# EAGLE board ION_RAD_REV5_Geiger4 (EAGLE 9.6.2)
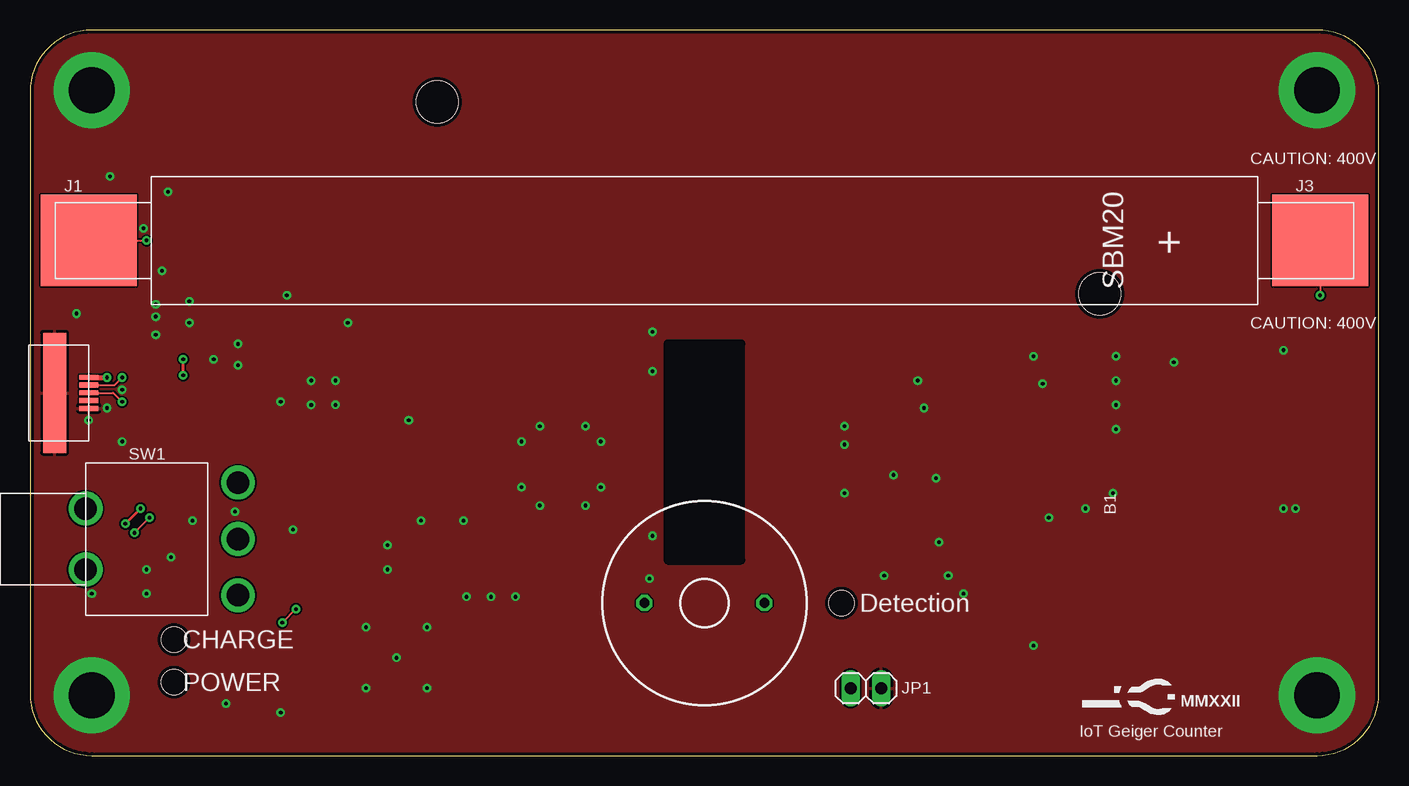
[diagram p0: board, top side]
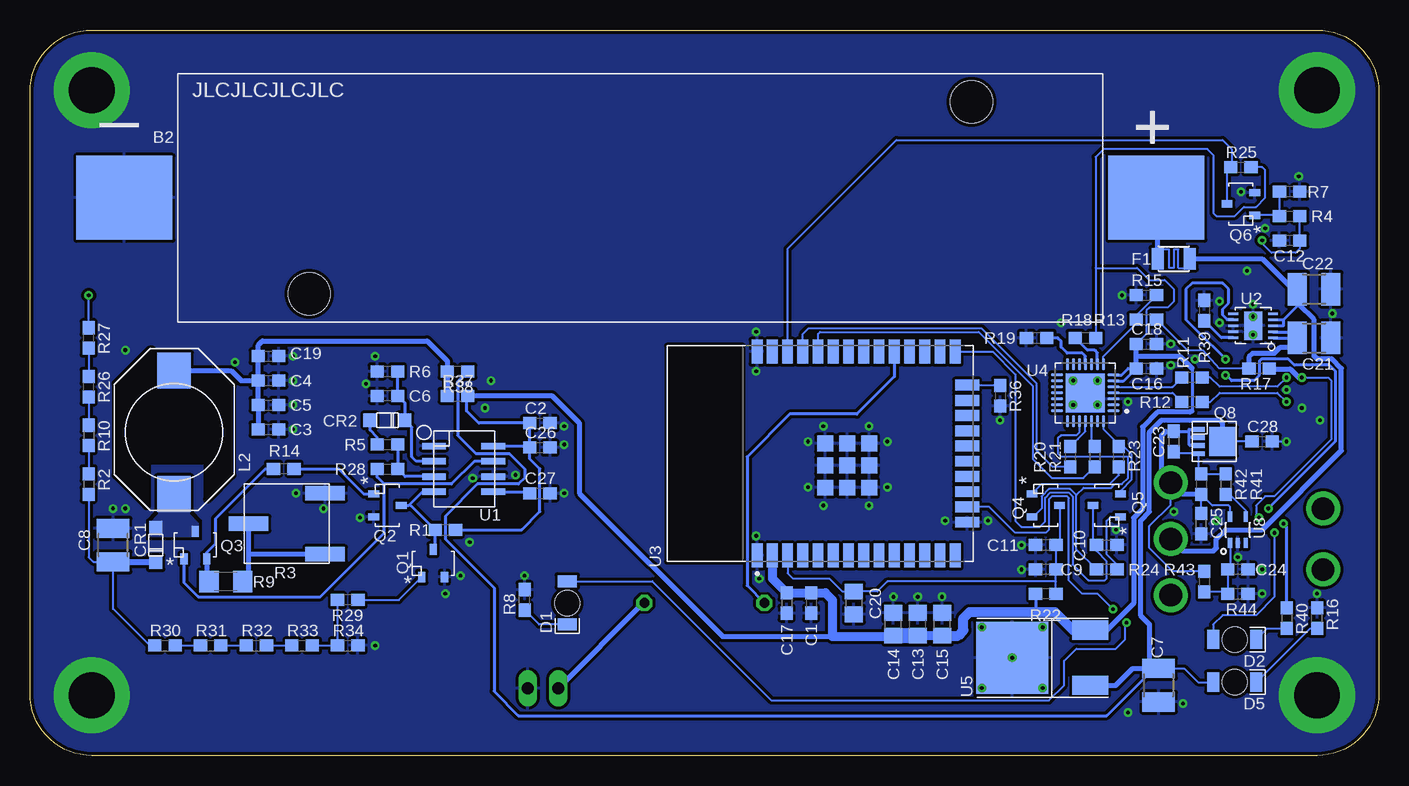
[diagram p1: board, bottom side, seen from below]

Size 112.4 x 60.5 mm. Coordinates in mm from the lower left corner, seen from the top.
Outline: 0,55.35 0,5.15 arc90 5.15,0 107.25,0 arc90 112.4,5.15 112.4,55.35 arc90 107.25,60.5 5.15,60.5 arc90 0,55.35
Copper layers (1*16): Top 0.035mm / dielectric 1.5mm / Bottom 0.035mm
Design rules "default *": minimum track width 6mil, minimum drill 12mil, track to track 6mil, track to pad 6mil, pad to pad 6mil, via to via 6mil, smd to smd 6mil, copper to edge 0.3mm, drill to drill 6mil, minimum pad ring 10mil, minimum via ring 8mil, stop-mask expansion 4mil, vias tented up to drill 12mil, thermal gap 10mil
Net classes: 1 HV: clearance 1.27 mm
tRestrict: area 53.2,16.3 to 59.2,34.3
bRestrict: area 95.6,20.9 to 105.2,33.8

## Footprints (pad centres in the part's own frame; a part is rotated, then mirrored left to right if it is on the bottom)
PS1740P02E = drill 0.813 octagon: 1 -5,0; 2 5,0
1042 = smd 8 x 7: + 43,0; - -43,0 | hole 3.5: -27.6,-8; 27.6,8
0603 = smd 1.1 x 1: 1 -0.85,0; 2 0.85,0
1210 = smd 1.6 x 2.7: 1 -1.4,0; 2 1.4,0
0805 = smd 1.3 x 1.5: 1 -0.95,0; 2 0.95,0
SOD123(AK) = smd 1.1 x 1.1: A 1.45,0; K -1.45,0
SOD123 = smd 1.1 x 1.1: 1 -1.45,0; 2 1.45,0
1206_REV = smd 1 x 1.6: A -1.8,0; K 1.8,0 | hole 2.1: 0,0
1206_FUSE_6M2_SS = smd 1.016 x 1.778: P$1 -1.333,0; P$2 1.333,0
01010002Z = smd 8.001 x 7.62: P$1 0,0
MICRO_USB = smd 0.4 x 1.6: 1 -1.3,0; 2 -0.65,0; 3 0,0; 4 0.65,0; 5 1.3,0 | smd 10 x 1.9: GND 0,-2.84
1X02 = drill 1.016 long: 1 -1.27,0; 2 1.27,0
SDR1005 = smd 3 x 2.8: P$1 -5.15,0; P$2 5.15,0
SOT23-3 = smd 0.6 x 0.9: 1 0.32,-1.15; 2 2.22,-1.15; 3 1.27,1.15
POWERPAK_1212-8 = smd 0.991 x 0.406: 1 -1.994,1.016; 2 -1.994,0.339; 3 -1.994,-0.339; 4 -1.994,-1.016 | smd 2.235 x 2.388: 15 0,0
3361P = smd 1.194 x 3.302: 1 -2.54,-3.188; 2 0,3.188; 3 2.54,-3.188
1206 = smd 1.6 x 1.8: 1 -1.4,0; 2 1.4,0
TOGGLE_RA = drill 1.88: 1 4.699,12.7; 2 0,12.7; 3 -4.699,12.7; P$4 -2.54,0; P$5 2.54,0
SOIC8 = smd 1.981 x 0.533: 1 -2.477,1.905; 2 -2.477,0.635; 3 -2.477,-0.635; 4 -2.477,-1.905; 5 2.477,-1.905; 6 2.477,-0.635; 7 2.477,0.635; 8 2.477,1.905
10DFN = smd 0.8 x 0.24: 1 -1.65,1; 2 -1.65,0.5; 3 -1.65,0; 4 -1.65,-0.5; 5 -1.65,-1; 6 1.65,-1; 7 1.65,-0.5; 8 1.65,0; 9 1.65,0.5; 10 1.65,1 | smd 1.5 x 2.4: GF 0,0
MODULE_ESP32-WROOM-32D = smd 2 x 0.9: 1 -8.5,5.26; 2 -8.5,3.99; 3 -8.5,2.72; 4 -8.5,1.45; 5 -8.5,0.18; 6 -8.5,-1.09; 7 -8.5,-2.36; 8 -8.5,-3.63; 9 -8.5,-4.9; 10 -8.5,-6.17; 11 -8.5,-7.44; 12 -8.5,-8.71; 13 -8.5,-9.98; 14 -8.5,-11.25; 25 8.5,-11.25; 26 8.5,-9.98; 27 8.5,-8.71; 28 8.5,-7.44; 29 8.5,-6.17; 30 8.5,-4.9; 31 8.5,-3.63; 32 8.5,-2.36; 33 8.5,-1.09; 34 8.5,0.18; 35 8.5,1.45; 36 8.5,2.72; 37 8.5,3.99; 38 8.5,5.26 | smd 0.9 x 2: 15 -5.715,-12.25; 16 -4.445,-12.25; 17 -3.175,-12.25; 18 -1.905,-12.25; 19 -0.635,-12.25; 20 0.635,-12.25; 21 1.905,-12.25; 22 3.175,-12.25; 23 4.445,-12.25; 24 5.715,-12.25 | smd 1.33 x 1.33: 39_1 -2.835,-0.405; 39_2 -1,-0.405; 39_3 0.835,-0.405; 39_4 -2.835,-2.24; 39_5 -1,-2.24; 39_6 0.835,-2.24; 39_7 -2.835,-4.075; 39_8 -1,-4.075; 39_9 0.835,-4.075
QFN50P500X500X80-29N = smd 1.01 x 0.27: 1 -2.36,1.5; 2 -2.36,1; 3 -2.36,0.5; 4 -2.36,0; 5 -2.36,-0.5; 6 -2.36,-1; 7 -2.36,-1.5; 15 2.36,-1.5; 16 2.36,-1; 17 2.36,-0.5; 18 2.36,0; 19 2.36,0.5; 20 2.36,1; 21 2.36,1.5 | smd 0.27 x 1.01: 8 -1.5,-2.36; 9 -1,-2.36; 10 -0.5,-2.36; 11 0,-2.36; 12 0.5,-2.36; 13 1,-2.36; 14 1.5,-2.36; 22 1.5,2.36; 23 1,2.36; 24 0.5,2.36; 25 0,2.36; 26 -0.5,2.36; 27 -1,2.36; 28 -1.5,2.36 | smd 3.25 x 3.25: 29 0,0
TO-252 = smd 1.6 x 3: 1 -2.3,-6.5; 3 2.3,-6.5 | smd 6 x 6: T 0,0
SC-70-5 = smd 0.85 x 0.35: 1 -1.1,0.65; 2 -1.1,0; 3 -1.1,-0.65; 4 1.1,-0.65; 5 1.1,0.65

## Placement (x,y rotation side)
B1  [PS1740P02E]  56.2,12.72 0 top
B2  1042  [1042]  61.53,46.51 0 bottom
C1  0.1uF  [0603]  47.31,12.72 270 bottom
C2  0.1uF  [0603]  69.92,27.71 0 bottom
C3  1uF  [0603]  92.52,27.2 0 bottom
C4  0.1uF  [0603]  92.52,31.27 0 bottom
C5  1uF  [0603]  92.52,29.23 0 bottom
C6  1nF  [0603]  82.62,30 180 bottom
C7  10uF  [1210]  18.35,5.87 270 bottom
C8  10nF 630V  [1210]  105.48,17.55 90 bottom
C9  0.1uF  [0603]  27.75,15.52 180 bottom
C10  0.1uF  [0603]  22.67,17.55 0 bottom
C11  0.1uF  [0603]  27.75,17.55 180 bottom
C12  100pF  [0603]  7.43,42.95 180 bottom
C13  10uF  [0805]  38.42,10.95 90 bottom
C14  1uF  [0805]  40.45,10.95 90 bottom
C15  1uF  [0805]  36.39,10.95 90 bottom
C16  0.1uF  [0603]  19.37,32.28 0 bottom
C17  0.1uF  [0603]  49.34,12.72 270 bottom
C18  0.1uF  [0603]  19.37,34.31 0 bottom
C19  1uF  [0603]  92.52,33.3 0 bottom
C20  10uF  [0805]  43.75,12.72 270 bottom
C21  4.7uF  [1210]  5.4,34.82 0 bottom
C22  4.7uF  [1210]  5.4,38.89 0 bottom
C23  0.1uF  [0603]  17.08,26.19 270 bottom
C24  0.1uF  [0603]  11.75,15.52 180 bottom
C25  0.1uF  [0603]  14.8,19.33 90 bottom
C26  0.1uF  [0603]  69.92,25.68 0 bottom
C27  0.1uF  [0603]  69.92,21.87 0 bottom
C28  0.1uF  [0603]  9.72,26.19 0 bottom
CR1  ES1JFL  [SOD123(AK)]  101.92,17.55 90 bottom
CR2  BAS21GWX  [SOD123]  82.62,27.96 180 bottom
D1  156120RS75300  [1206_REV]  67.63,12.72 270 bottom
D2  156120RS75300  [1206_REV]  12,9.68 0 bottom
D5  156120RS75300  [1206_REV]  12,6.12 0 bottom
F1  1206_FUSE6M2SS  [1206_FUSE_6M2_SS]  17.08,41.43 0 bottom
J1  01010002Z  [01010002Z]  4.89,42.95 0 top
J3  01010002Z  [01010002Z]  107.51,42.95 0 top
J7  10104110-0001LF  [MICRO_USB]  4.89,30.25 270 top
JP1  [1X02]  69.66,5.61 0 top
L2  10mH  [SDR1005]  100.4,26.95 90 bottom
Q1  MMBT3904  [SOT23-3]  80.08,16.03 0 bottom
Q2  MMBT3904  [SOT23-3]  82.62,22.12 270 bottom
Q3  PMBTA45,215  [SOT23-3]  99.89,17.55 0 bottom
Q4  MMBT3904  [SOT23-3]  27.75,22.12 270 bottom
Q5  MMBT3904  [SOT23-3]  22.67,19.58 90 bottom
Q6  MMBT3904  [SOT23-3]  11.5,44.73 90 bottom
Q8  SIS413DN-T1-GE3  [POWERPAK_1212-8]  13.02,26.19 0 bottom
R1  100k  [0603]  77.79,18.82 0 bottom
R2  1M  [0603]  107.51,22.63 270 bottom
R3  10  [3361P]  91,19.33 90 bottom
R4  20k  [0603]  7.43,44.98 0 bottom
R5  1k  [0603]  82.62,25.93 0 bottom
R6  220k  [0603]  82.62,32.03 0 bottom
R7  100k  [0603]  7.43,47.01 180 bottom
R8  499  [0603]  71.19,12.98 90 bottom
R9  10  [1206]  96.08,14.5 180 bottom
R10  1M  [0603]  107.51,26.69 270 bottom
R11  10  [0603]  15.56,31.52 180 bottom
R12  10  [0603]  15.56,29.49 180 bottom
R13  22.1k  [0603]  19.37,36.35 0 bottom
R14  10  [0603]  91.25,23.9 180 bottom
R15  47.5k  [0603]  19.37,38.38 0 bottom
R16  10k  [0603]  5.15,11.45 90 bottom
R17  0  [0603]  9.97,32.28 180 bottom
R18  1k  [0603]  24.45,34.82 0 bottom
R19  10k  [0603]  28.51,34.82 0 bottom
R20  0  [0603]  25.72,24.92 270 bottom
R21  0  [0603]  23.69,24.92 270 bottom
R22  1k  [0603]  27.75,13.49 180 bottom
R23  10k  [0603]  21.66,24.92 90 bottom
R24  10k  [0603]  22.67,15.52 180 bottom
R25  10k  [0603]  11.5,49.05 0 bottom
R26  1M  [0603]  107.51,30.76 90 bottom
R27  1M  [0603]  107.51,34.82 90 bottom
R28  330  [0603]  82.62,23.9 0 bottom
R29  10  [0603]  85.92,12.98 180 bottom
R30  3.3M  [0603]  101.16,9.17 0 bottom
R31  3.3M  [0603]  97.35,9.17 0 bottom
R32  3.3M  [0603]  93.54,9.17 0 bottom
R33  3.3M  [0603]  89.73,9.17 0 bottom
R34  20k  [0603]  85.92,9.17 0 bottom
R36  10k  [0603]  31.56,30 270 bottom
R37  DNP  [0603]  76.77,30 0 bottom
R38  0  [0603]  76.77,32.03 0 bottom
R39  2k  [0603]  14.54,37.11 270 bottom
R40  1k  [0603]  7.69,11.45 270 bottom
R41  1k  [0603]  12.77,22.63 270 bottom
R42  100k  [0603]  14.8,22.63 270 bottom
R43  1k  [0603]  14.54,14.5 270 bottom
R44  1k  [0603]  11.75,13.49 0 bottom
SW1  SPDT  [TOGGLE_RA]  4.64,18.06 270 top
T1  SBM-20  [SBM-20]  56.2,42.95 0 top
U1  TLC555CDG4  [SOIC8]  76.27,23.9 0 bottom
U2  MCP73114-0NSI/MF  [10DFN]  10.48,35.84 180 bottom
U3  ESP32-WROOM-32D  [MODULE_ESP32-WROOM-32D]  46.55,25.17 90 bottom
U4  CP2102N-A01-GQFN28  [QFN50P500X500X80-29N]  24.45,30.25 180 bottom
U5  UA78M33CKVURG3  [TO-252]  30.55,8.15 90 bottom
U8  MIC842LYC5-TR  [SC-70-5]  11.75,18.82 90 bottom

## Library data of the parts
B1 = mightyohm; OC_FARNELL: unknown; OC_NEWARK: unknown
B2 = ruark2; PARTNO: 36-1042-ND
C1-C28 F1 R1 R2 R4-R34 R36-R44 T1 U8 = ruark2
CR1 = ruark2; PARTNO: ES1JFLCT-ND
CR2 = ruark2; PARTNO: 1727-7323-1-ND
D1 D2 D5 = ruark2; PARTNO: 732-5031-1-ND
J1 J3 = ruark2; PARTNO: F4080-ND
J7 = ruark2; PARTNO: 609-4052-1-ND
JP1 = pinhead
L2 = ruark2; PARTNO: SDR1005-103KLCT-ND
Q1 Q2 Q4-Q6 = ruark2; PARTNO: MMBT3904TPMSCT-ND
Q3 = ruark2; PARTNO: 1727-5332-1-ND
Q8 = ruark2; PARTNO: SIS413DN-T1-GE3CT-ND
R3 = ruark2; PARTNO: 3361P-1-100GLFCT-ND
SW1 = ruark2; PARTNO: EG2362-ND
U1 = ruark2; PARTNO: 296-52992-ND
U2 = ruark2; PARTNO: MCP73114-0NSI/MF-ND
U3 = ESP32-WROOM-32D; AVAILABILITY: Bad; DESCRIPTION: Bluetooth, WiFi 802.11b/g/n, Bluetooth v4.2 +EDR, Class 1, 2 and 3 Transceiver Module 2.4GHz ~ 2.5GHz Integrated, Trace Surface Mount; MF: Espressif Systems; MP: ESP32-WROOM-32D; PACKAGE: Module Espressif Systems; PRICE: None
U4 = CP2102N-A01-GQFN28; AVAILABILITY: In Stock; DESCRIPTION: USB Bridge, USB to UART USB 2.0 UART Interface 28-QFN (5x5); MF: Silicon Labs; MP: CP2102N-A01-GQFN28; PACKAGE: WFQFN-28 Silicon Labs; PRICE: None
U5 = ruark2; PARTNO: 296-21208-1-ND

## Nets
+3V3: C1.1 C2.1 C13.1 C14.1 C15.1 C16.1 C17.1 C18.1 C26.1 R1.2 R18.2 R22.2 R25.2 R37.2 U1.8 U3.2 U4.6 U4.7 U5.3
+5V: C7.1 C28.1 D5.A Q8.15 R38.2 U5.1
DTR: Q5.2 R23.2 U4.28
EN: C9.1 C11.1 C20.1 Q4.3 R22.1 U3.3
GM_PULSE: Q6.3 R25.1 U3.36
GND: B2.- C1.2 C2.2 C3.2 C4.2 C5.2 C6.2 C7.2 C8.2 C9.2 C10.2 C11.2 C12.2 C13.2 C14.2 C15.2 C16.2 C17.2 C18.2 C19.2 C20.2 C21.2 C22.2 C24.1 C25.1 C26.2 C27.2 C28.2 J7.5 J7.GND JP1.2 Q1.2 Q2.2 Q6.2 R3.3 R6.1 R7.1 R8.2 R15.1 R16.2 R19.1 R34.2 R36.2 R39.1 R44.2 U1.1 U1.6 U2.8 U2.9 U2.GF U3.1 U3.15 U3.38 U3.39_1 U3.39_2 U3.39_3 U3.39_4 U3.39_5 U3.39_6 U3.39_7 U3.39_8 U3.39_9 U4.3 U4.29 U5.T U8.2
HV [HV]: C8.1 CR1.K R2.2 R30.1
IO0: C10.1 Q5.3 U3.25
IO2: R36.1 U3.24
IO4: U3.26
IO16: U3.27
IO17: U3.28
IO18: U3.30
IO19: U3.31
LED: D1.A U3.16
N$1: CR2.2 R5.1
N$2: J7.2 R11.1
N$3: Q1.3 Q2.3 R1.1 U1.4
N$4: J7.3 R12.1
N$5: R11.2 U4.5
N$6: R12.2 U4.4
N$7: R13.1 R15.2 U4.8
N$8: Q3.1 R28.1 U1.7
N$9: C6.1 CR2.1 R6.2 U1.2
N$10: R5.2 R28.2 U1.3
N$11: Q3.2 R9.2 R14.2
N$12: B1.2 JP1.1
N$14: Q6.1 R4.1 R7.2
N$15 [HV]: J3.P$1 R27.2
N$16 [HV]: R2.1 R10.2
N$17 [HV]: R10.1 R26.1
N$18: R18.1 U4.9
N$19: D5.K R16.1
N$20: R19.2 U4.11
N$21 [HV]: R26.2 R27.1
N$22: Q4.1 R23.1
N$23: R3.1 R3.2 R9.1
N$24: Q5.1 R24.1
N$25: Q2.1 R14.1
N$26: Q1.1 R29.1
N$27: D1.K R8.1
N$28 [HV]: R31.2 R32.1
N$29: R29.2 R33.2 R34.1
N$30 [HV]: R30.2 R31.1
N$31 [HV]: R32.2 R33.1
N$32: B2.+ F1.P$1
N$33: C27.1 U1.5
N$34: R40.1 U2.7
N$35: C3.1 C4.1 C5.1 C19.1 L2.P$2 R37.1 R38.1
N$37: D2.K R40.2
N$39: C12.1 J1.P$1 R4.2
N$40: R41.2 U8.4
N$41: R39.2 U2.10
N$42: C22.1 F1.P$2 SW1.2 U2.3 U2.4
N$44: C23.2 Q8.4 R41.1 R42.1
N$46: C23.1 C25.2 Q8.1 Q8.2 Q8.3 R42.2 R43.1 SW1.3 U8.5
N$47: C24.2 R43.2 R44.1 U8.1
PIEZO: B1.1 U3.29
RTS: Q4.2 R24.2 U4.24
RXD: R20.1 U4.25
RXD0: R21.2 U3.34
SW [HV]: CR1.A L2.P$1 Q3.3
TXD: R21.1 U4.26
TXD0: R20.2 U3.35
VUSB: C21.1 R13.2 R17.2 U2.1 U2.2
VUSBIN: D2.A J7.1 R17.1

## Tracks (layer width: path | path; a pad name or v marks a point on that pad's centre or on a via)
+3V3
  Bottom 0.152: R25.2 9.72,49.05 9.46,48.79 9.46,46.51 10.23,45.74 11.24,45.74 12,44.98 13.53,44.98 13.78,45.24 13.78,50.06 14.29,50.57 22.93,50.57 23.6,49.9 23.6,40.66 | 23.6,40.66 R18.2 | 23.6,40.66 20.13,40.66 19.12,39.65 17.85,39.65 17.08,38.89 17.08,37.87 17.59,37.36 19.11,37.36 19.37,37.1 19.37,35.16 C18.1
  Bottom 0.254: U4.6 21.25,31.25 C16.1 20.89,32.28 21.43,31.75 U4.7 | U1.8 70.89,25.8 C26.1 | C26.1 C2.1 75,27.71 76.01,28.73 76.01,29.91 R37.2 | R1.2 71.44,18.82 69.92,20.34 69.92,23.9 70.77,24.75 C26.1 | 15.56,32.28 15.56,28.73 | R22.2 28.6,12.05 28.51,11.96
  Bottom 0.406: C16.1 20.22,33.3 | 20.22,33.3 C18.1 | R37.2 68.9,30 66.61,27.71 66.61,21.87 54.68,9.93 45.53,9.93 | 20.22,33.3 16.58,33.3 15.56,32.28 | 15.56,28.73 15.62,28.73 15.71,28.63 18.45,28.63 19.68,27.41 19.68,20.57 20.44,19.81 20.44,12.67 22.66,10.45 23.43,10.45 U5.3
  Bottom 0.762: U3.2 50.54,14.77 C17.1 C1.1 46.13,13.57 45.53,12.98 45.53,9.93 40.52,9.93 C14.1 | C15.1 C13.1
  Bottom 0.813: C15.1 35.05,10 34.61,10.44 34.61,11.45 34.1,11.96 28.51,11.96 26.99,11.96 25.48,10.45 23.43,10.45
  Bottom 1.27: C13.1 C14.1
+5V
  Bottom 0.152: C28.1 Q8.15 | C7.1 17.85,7.27 16.2,7.27 15.05,6.12 D5.A
  Bottom 0.254: R38.2 76.77,31.18 76.77,26.69 75.25,25.17 72.46,25.17 71.19,23.9 71.19,23.14 71.69,22.63 75.11,22.63 77.79,19.95 77.79,18.06 73.73,13.99 73.73,5.36 71.69,3.33 22.67,3.33 18.67,7.33 18.42,7.33
  Bottom 0.406: Q8.15 13.02,27.71 13.27,27.96 18.1,27.96 19.12,26.95 19.12,20.34 19.88,19.58 19.88,11.71 19.12,10.95 19.12,8.03 18.42,7.33 C7.1 | U5.1 21.92,5.85 20.51,7.27 17.85,7.27
DTR
  Bottom 0.152: U4.28 22.95,27.23 21.66,25.93 R23.2 21.24,25.77 20.59,25.12 20.59,23.01 21.52,22.08 Q5.2
EN
  Bottom 0.152: Q4.3 26.6,17.85 C11.1 C9.1 26.9,14.5 | R22.1 26.9,14.5 | 26.9,14.5 40.96,14.5 41.79,13.67 C20.1 44.7,13.67 45.79,14.76 48.83,14.76 49.27,15.19 U3.3
GM_PULSE
  Bottom 0.152: Q6.3 12.65,48.75 R25.1 12.26,49.13 12.26,50.57 13.02,51.33 40.2,51.33 49.27,42.26 U3.36
GND  (via drill 0.3, 3.81 pad 6.35)
  Bottom 0.152: C28.2 v7.69,26.19
  Bottom 0.406: U4.29 v25.47,29.23
  other vias: 5.15,55.48 5.15,5.02 107.25,55.48 107.25,5.02 21.91,18.82 84.9,19.84 71.95,23.39 67.88,25.93 84.39,31.01 83.63,33.3 90.49,31.27 104.46,20.6 105.48,20.6 11.5,47.01 6.67,48.28 9.46,43.97 25.47,31.27 23.43,29.23 23.43,31.27 20.89,29.49 17.34,34.31 17.34,32.54 29.78,17.55 29.78,15.52 21.4,38.38 4.89,27.96 26.48,36.09 75.5,23.14 75.76,17.8 40.45,13.23 38.42,13.23 36.39,13.23 33.09,10.69 20.89,3.58 7.69,30.5 11.75,16.53 9.72,15.52 13.53,19.58 17.08,20.34 9.72,13.49 5.15,13.49 15.31,33.04 10.99,40.41 3.88,36.85 67.88,27.46 67.88,21.87 36.13,19.58 32.58,19.58 42.48,20.85 51.63,14.76 51.88,18.31 51.88,32.03 51.88,35.33 40.96,22.38 40.96,26.19 42.48,27.46 46.29,27.46 47.56,26.19 47.56,22.38 46.29,20.85 31.56,27.96 6.42,28.98 83.63,9.17 77.79,13.49 76.52,15.01 71.19,15.01 16.32,4.34 90.49,29.23 90.49,27.2 90.24,21.87 87.95,20.6 95.32,32.79 104.46,33.81 73.98,31.27 74.49,28.98 13.27,36.09 10.48,35.08 10.48,36.6 10.48,37.62 13.27,37.87 28.01,10.69 33.09,5.61 28.01,5.61 30.55,8.15 90.49,33.3
  pour Top: 0.2,54.25 0.2,55.1 arc-90 5.35,60.25 107.05,60.25 arc-90 112.2,55.1 112.2,5.4 arc-90 107.05,0.25 5.35,0.25 arc-90 0.2,5.4
  pour Bottom (isolate 0.254, rank 4): 0.2,54.25 0.2,55.1 arc-90 5.35,60.25 107.05,60.25 arc-90 112.2,55.1 112.2,5.4 arc-90 107.05,0.25 5.35,0.25 arc-90 0.2,5.4
  pour Bottom: 109.84,16.89 109.84,36.04 111.06,36.04 111.06,19.43
HV
  Bottom 0.152: 104.08,16.15 105.22,16.15 C8.1 105.48,12.22 102.43,9.17 R30.1 | R2.2 107.51,16.53 107.12,16.15 105.73,16.15
  Bottom 0.406: 106.49,16.28 106.36,16.15 105.73,16.15 C8.1
  Bottom 0.508: CR1.K 105.17,16.1 105.22,16.15
IO0
  Bottom 0.152: Q5.3 23.82,17.85 C10.1 23.52,17.04 22.67,16.19 22.67,14.76 22.82,14.61 24.2,14.61 25.52,15.93 25.52,21.59 25.85,21.92 27.37,21.92 27.8,21.49 27.8,19.53 28.26,19.07 29.78,19.07 30.29,19.58 30.29,31.77 32.19,33.67 U3.25
IO2
  Bottom 0.152: U3.24 31.6,30.89 R36.1
LED  (via drill 0.3)
  Top 0.152: v21.03,11.08 v22.16,12.22
  Bottom 0.152: D1.A 60.54,14.52 50.61,4.6 27.5,4.6 26.23,5.87 26.23,7.9 25.21,8.91 21.91,8.91 21.15,9.68 21.15,11.2 v21.03,11.08 | U3.16 32.45,20.73 30.29,18.57 27.75,18.57 27.5,18.82 27.5,21.36 27.24,21.61 25.97,21.61 25.82,21.46 25.82,15.52 25.82,14.6 24.7,13.49 23.43,13.49 v22.16,12.22
N$1
  Bottom 0.254: R5.1 83.47,26.53 84.07,27.13 CR2.2
N$2  (via drill 0.3)
  Top 0.152: J7.2 7.07,30.9 v7.69,31.52
  Bottom 0.152: v7.69,31.52 8.45,30.76 13.27,30.76 14.04,31.52 R11.1
N$3
  Bottom 0.254: 78.87,21.87 U1.4 79.7,21.99 80.84,20.85 | Q2.3 80.84,20.85 | 80.84,20.85 80.67,20.85 R1.1 78.64,17.34 Q1.3
N$4  (via drill 0.3)
  Top 0.152: J7.3 6.92,30.25 v7.69,29.49
  Bottom 0.152: R12.1 14.04,29.49 13.27,30.25 8.45,30.25 v7.69,29.49
N$5
  Bottom 0.152: U4.5 17.18,30.75 R11.2
N$6
  Bottom 0.152: U4.4 17.17,30.25 R12.2
N$7
  Bottom 0.152: U4.8 22.95,33.27 20.22,36 R13.1 20.22,36.68 R15.2
N$8
  Bottom 0.254: U1.7 75.38,24.54 77.28,22.63 82.87,22.63 | R28.1 83.47,23.23 82.87,22.63 | Q3.1 99.57,14.44 98.36,13.23 88.2,13.23 82.87,18.57 82.87,22.63
N$9
  Bottom 0.254: U1.2 80.2,24.54 80.58,24.92 80.58,27.38 CR2.1 81.17,29.4 C6.1 R6.2
N$10
  Bottom 0.254: U1.3 81.13,23.27 R28.2 R5.2
N$11
  Bottom 0.254: Q3.2 97.67,16.92 96.92,17.67 96.92,19.76 92.78,23.9 R14.2
  Bottom 0.406: Q3.2 97.67,14.69 R9.2
N$12
  Bottom 0.406: JP1.1 61.28,12.72 B1.2
N$14
  Bottom 0.152: R7.2 R4.1 8.35,45.05 Q6.1
N$15  (via drill 0.3)
  Top 0.152: J3.P$1 v107.51,38.38
  Bottom 0.152: R27.2 v107.51,38.38
N$16
  Bottom 0.152: R10.2 R2.1
N$17
  Bottom 0.152: R26.1 R10.1
N$18
  Bottom 0.254: U4.9 23.45,33.57 23.69,33.81 24.28,33.81 R18.1
N$19
  Bottom 0.152: D5.K 5.72,10.6 R16.1
N$20
  Bottom 0.254: U4.11 24.45,33.3 24.7,33.55 25.97,33.55 26.48,34.06 26.48,34.57 26.74,34.82 R19.2
N$21
  Bottom 0.152: R27.1 R26.2
N$22
  Bottom 0.152: R23.1 21.66,23.39 22.42,22.63 28.07,22.63 Q4.1
N$23
  Bottom 0.406: 94.81,14.37 R9.1 94.19,14.99 94.19,16.79 | 94.19,16.79 R3.2 | R3.1 94.19,16.79
N$24
  Bottom 0.152: R24.1 21.82,15.94 22.67,16.79 22.67,19.58 22.35,19.9 Q5.1
N$25
  Bottom 0.254: R14.1 86.68,23.9 84.58,21.8 Q2.1
N$26
  Bottom 0.152: R29.1 81.65,12.98 Q1.1
N$27
  Bottom 0.152: D1.K 69.98,10.92 R8.1
N$28
  Bottom 0.152: R31.2 R32.1
N$29
  Bottom 0.152: R33.2 R34.1 R29.2
N$30
  Bottom 0.152: R30.2 R31.1
N$31
  Bottom 0.152: R32.2 R33.1
N$32
  Bottom 0.406: F1.P$1 18.42,47.08 18.53,47.19 | 18.86,47.52 18.53,47.19 | 18.53,47.19 B2.+
N$33
  Bottom 0.254: U1.5 70.89,21.99 C27.1
N$34  (via drill 0.3)
  Top 0.254: v7.94,19.33 v9.21,20.6 | v12.77,31.7 v12.77,33.04
  Bottom 0.254: R40.1 7.69,19.07 v7.94,19.33 | v9.21,20.6 3.6,26.21 3.6,32.03 4.13,32.56 7.04,32.56 7.54,33.06 9.79,33.06 9.95,32.9 9.95,31.8 9.99,31.75 9.99,31.67 10.39,31.27 12.26,31.27 12.77,31.77 v12.77,31.7 | U2.7 12.63,36.35 13.02,36.74 13.02,37.23 12.51,37.73 12.51,38.89 13.02,39.39 15.56,39.39 16.07,38.89 16.07,36.34 15.16,35.43 15.15,35.43 v12.77,33.04
N$35
  Bottom 0.406: L2.P$2 95.64,32.1 94.81,31.27 C4.1 | C4.1 C5.1 C3.1 | C4.1 C19.1 93.37,34.23 93.03,34.57 79.31,34.57 77.62,32.88 R38.1 R37.1
N$37
  Bottom 0.152: D2.K 9.28,10.6 R40.2
N$39  (via drill 0.3)
  Top 0.152: J1.P$1 v9.72,42.95
  Bottom 0.152: R4.2 C12.1 6.58,42.28 6.92,41.93 8.96,41.93 9.72,42.7 v9.72,42.95
N$40
  Bottom 0.152: R41.2 12.42,21.78 11.1,20.46 U8.4
N$41
  Bottom 0.254: U2.10 13.12,34.84 R39.2
N$42
  Bottom 0.254: U2.3 7.94,35.84 7.94,36.35 | C22.1 6.67,38.76 6.67,37.62 7.94,36.35 | U2.4 7.95,36.34 7.94,36.35
  Bottom 0.406: SW1.2 16.32,17.04 13.78,17.04 13.53,17.3 13.53,18.06 12.77,18.82 9.72,18.82 3.11,25.42 3.11,32.28 3.88,33.04 5.15,33.04 5.4,33.3 5.4,36.35 6.67,37.62 | C22.1 7.18,38.89 9.72,41.43 F1.P$2
N$44
  Bottom 0.152: C23.2 16.92,25.17 Q8.4 15.01,23.7 R42.1 R41.1
N$46
  Bottom 0.152: 14.54,15.77 R43.1 17.17,15.35 19.12,17.3 19.12,19.14 17.34,20.92 SW1.3 | C25.2 R42.2 13.87,20.85 12.51,20.85 12.4,20.74 U8.5
  Bottom 0.254: Q8.3 15.73,25.85 15.81,25.93 15.81,26.44 | 15.81,26.44 15.81,26.95 | 15.81,26.95 15.81,27.2 Q8.1 | Q8.2 15.73,26.52 15.81,26.44 | C23.1 15.9,27.04 15.81,26.95
  Bottom 0.406: R42.2 16.36,21.78 SW1.3 18.1,23.52 18.1,26.69 17.76,27.04 C23.1
N$47
  Bottom 0.152: R43.2 12.77,13.65 R44.1 C24.2 | 12.91,15.83 C24.2 | U8.1 12.4,15.72 C24.2
PIEZO
  Bottom 0.254: U3.29 40.38,31.59 43.5,28.47 49.09,28.47 52.64,24.92 52.64,14.17 B1.1
RTS
  Bottom 0.152: R24.2 25.21,17.21 25.21,21.71 | U4.24 24.96,26.95 25.21,26.69 26.48,26.69 26.74,26.44 26.74,25.17 26.48,24.92 20.89,24.92 20.89,23.14 21.4,22.63 21.99,22.63 22.29,22.32 24.6,22.32 25.21,21.71 | Q4.2 28.8,19.9 28.11,20.6 28.11,21.61 27.5,22.22 25.72,22.22 25.21,21.71
RXD
  Bottom 0.152: R20.1 25.26,26.23 25.21,26.27 25.1,26.39 25.09,26.39 24.45,27.02 U4.25
RXD0
  Bottom 0.152: R21.2 24.62,23.14 27.24,23.14 28.82,24.71 28.82,30.81 33.34,35.33 46.55,35.33 46.73,35.15 U3.34
SW
  pour Bottom (no thermals): 102.43,19.33 102.43,18.31 98.36,18.31 98.36,19.33 99.13,20.09 99.13,23.14 101.67,23.14 101.67,20.09
TXD
  Bottom 0.152: U4.26 23.95,26.03 R21.1
TXD0
  Bottom 0.152: R20.2 arc90 25.89,23.9 | 26.06,24.41 R20.2 | U3.35 48,35.15 47.51,35.63 33.14,35.63 28.51,31.01 28.51,25.42 27.16,24.07 R20.2
VUSB
  Bottom 0.152: R13.2 15.98,33.81 14.69,33.81 13.31,32.28 R17.2
  Bottom 0.254: U2.2 7.18,35.33 6.8,34.95 C21.1 8.81,34.82 U2.1
  Bottom 0.406: 10.89,32.22 R17.2 10.82,33.21 10.48,33.55 8.7,33.55 8.19,34.06 6.42,34.06 6.42,34.57 6.8,34.95
VUSBIN  (via drill 0.3)
  Top 0.152: v9.97,19.84 v8.7,18.57
  Top 0.406: J7.1 4.92,31.52 v6.42,31.52
  Bottom 0.152: v6.42,31.52 4.21,31.52 3.95,31.27 3.95,26.36 8.7,21.61 9.46,21.61 10.23,20.85 10.23,20.09 v9.97,19.84 | v8.7,18.57 8.7,13.23 10.23,11.71 13.02,11.71 13.8,10.92 D2.A
  Bottom 0.406: R17.1 9.07,32.23 7.39,32.23 6.68,31.52 v6.42,31.52

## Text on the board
tPlace: CAUTION: 400V | CAUTION: 400V | MMXXII | IoT Geiger Counter
tNames: Detection | CHARGE | POWER
bNames: JLCJLCJLCJLC
tStop: 036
